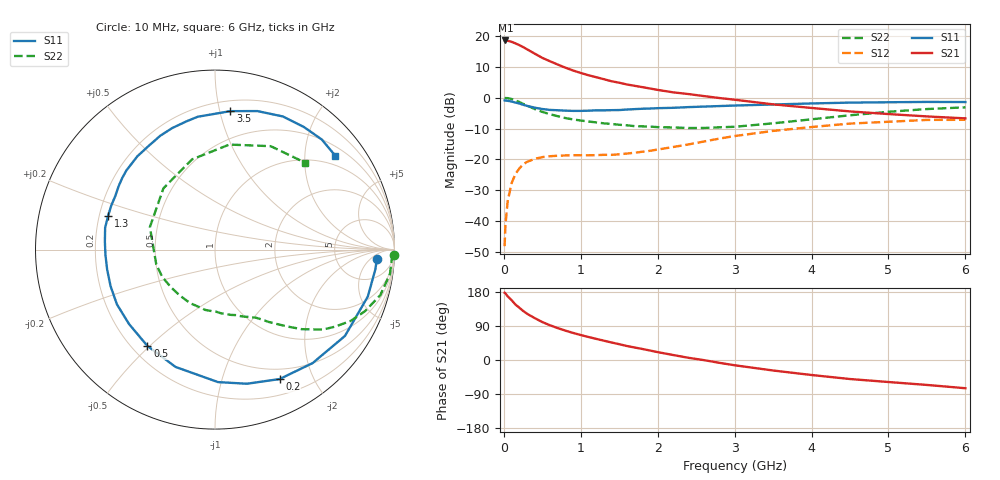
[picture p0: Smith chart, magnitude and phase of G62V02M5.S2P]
! SIEMENS Small Signal Semiconductors
! BFG193
! Si NPN RF Bipolar Junction Transistor in SOT223
! VCE = 2 V  IC = 2.5 mA
! Common Emitter S-Parameters:  August  1996
# GHz  S  MA  R  50
!  f  S11  S21  S12  S22
! GHz  MAG  ANG  MAG  ANG  MAG  ANG  MAG  ANG
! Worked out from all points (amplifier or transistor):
!   36 points, 10 MHz to 6 GHz, reference 50 ohm
!   highest |S21| = 18.6 dB at 20 MHz (marker M1)
!   |S21| within 3 dB of that: start of sweep to 311.1 MHz
!   unconditionally stable (mu >= 1): 1.31 GHz to 2.692 GHz
!   at 250 MHz: K = 0.21, MSG = 19.1 dB, |S12| = -21.7 dB
!   at 1.4 GHz: K = 1.07, MAG = 10.3 dB, |S12| = -18.6 dB
!   at 6 GHz: K = 0.96, MSG = 0.2 dB, |S12| = -7.2 dB
!   S11 on the Smith chart (normalised r, x): 10 MHz: 15, -9; 200 MHz: 0.38, -1.55; 500 MHz: 0.26, -0.49; 1.3 GHz: 0.24, +0.14; 3.5 GHz: 0.28, +1.08; 6 GHz: 0.72, +2.73
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0.01  0.9035 -3.4  8.423 177.5  0.0039 87.7  0.9951 -1.6
0.02  0.9001 -7.1  8.491 176.2  0.0083 88.9  0.9865 -3.1
0.05  0.8907 -17.1  8.395 167.8  0.021 80.1  0.9842 -8.0
0.1  0.8693 -33.6  8.073 158.1  0.0409 72.5  0.9552 -15.4
0.15  0.8341 -49.3  7.62 146.5  0.0574 63.0  0.9037 -22.3
0.2  0.806 -63.5  7.145 138.2  0.0708 56.7  0.8542 -27.7
0.25  0.7683 -76.6  6.638 129.7  0.0824 50.3  0.796 -32.6
0.3  0.7384 -88.7  6.121 122.3  0.0908 45.3  0.7476 -36.6
0.4  0.6897 -108.6  5.197 110.7  0.1018 37.1  0.6563 -42.5
0.5  0.6556 -125.1  4.431 100.1  0.1086 31.1  0.5889 -46.7
0.6  0.6334 -139.2  3.902 91.7  0.1124 27.2  0.5397 -50.2
0.7  0.6258 -150.9  3.454 84.2  0.1143 24.5  0.501 -53.5
0.9  0.6111 -169.6  2.765 71.4  0.1168 21.2  0.4444 -58.8
1.1  0.6153 175.7  2.315 60.7  0.1165 20.4  0.4107 -65.6
1.3  0.6244 162.7  1.997 51.0  0.1183 21.2  0.3836 -72.1
1.6  0.6428 146.6  1.639 36.9  0.1242 24.1  0.3563 -84.7
2.2  0.6856 122.7  1.223 13.2  0.1585 27.8  0.3291 -114.8
2.8  0.7317 102.7  0.989 -7.4  0.2168 23.7  0.331 -152.5
3.5  0.776 83.7  0.78 -27.7  0.2893 9.5  0.3839 160.9
4.5  0.8326 63.0  0.599 -50.2  0.3803 -12.8  0.5187 104.3
5.5  0.8545 45.9  0.497 -65.8  0.4363 -39.8  0.6545 61.7
6  0.8503 38.0  0.462 -74.5  0.4378 -54.5  0.6984 43.8
